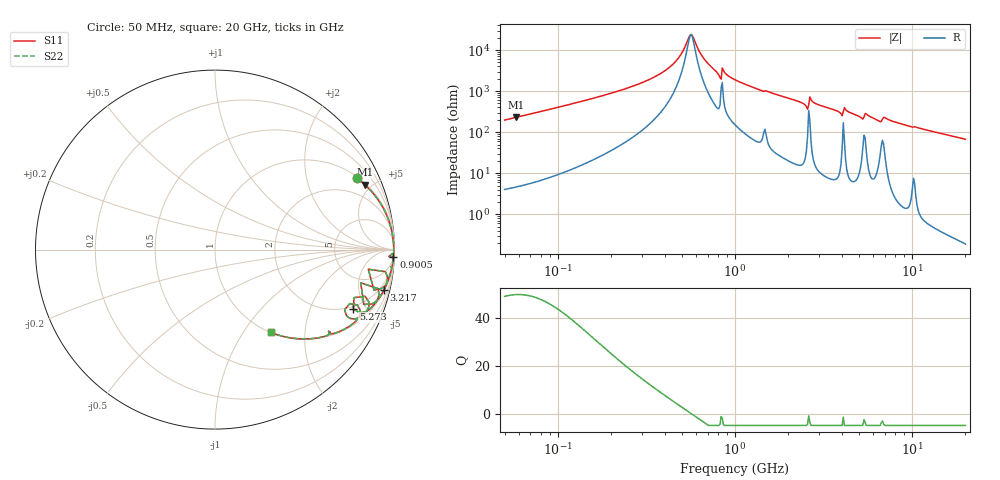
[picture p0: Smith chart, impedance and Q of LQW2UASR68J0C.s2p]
!Murata Part Number: LQW2UASR68J0C
!These Parameters are Measured in Series Mode Connection
!  o--[Z]--o
!Port1  Port2
!  o-------o
!Freq. Start=50[MHz] Stop=20[GHz], 401[Steps]
# Hz S RI R 50
!Freq.(Hz) S11(Real) S11(Imag) S21(Real) S21(Imag) S12(Real) S12(Imag) S22(Real) S22(Imag)
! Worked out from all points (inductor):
!   401 points, 50 MHz to 20 GHz, reference 50 ohm
!   read as one part in series: L = 621 nH near 51.52 MHz
!   highest Q = 49.8 at 58.08 MHz (marker M1), where L = 628 nH
!   self-resonance near 557.6 MHz
!   S11 on the Smith chart (normalised r, x): 50 MHz: 1.08, +3.94; 900.5 MHz: 7, -49; 3.217 GHz: 1.17, -8.26; 5.273 GHz: 1.84, -4.09; 20 GHz: 1.00, -1.34
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5e7  0.7903 0.397  0.2097 -0.397  0.2097 -0.397  0.7903 0.397
5.807932e7  0.8353 0.361  0.1647 -0.361  0.1647 -0.361  0.8353 0.361
1.364002e8  0.9652 0.1699  0.0348 -0.1699  0.0348 -0.1699  0.9652 0.1699
2.520729e8  0.9892 0.0803  0.0108 -0.0803  0.0108 -0.0803  0.9892 0.0803
3.721004e8  0.9943 0.0387  0.00569 -0.0387  0.00569 -0.0387  0.9943 0.0387
4.658406e8  0.9955 0.0175  0.00446 -0.0175  0.00446 -0.0175  0.9955 0.0175
5.659842e8  0.9959 -0.000196  0.00414 0.000196  0.00414 0.000196  0.9959 -0.000196
6.574395e8  0.9956 -0.014  0.00435 0.014  0.00435 0.014  0.9956 -0.014
8.108264e8  0.9924 -0.0394  0.00762 0.0394  0.00762 0.0394  0.9924 -0.0394
8.738837e8  0.9936 -0.0344  0.00636 0.0344  0.00636 0.0344  0.9936 -0.0344
9.00459e8  0.9939 -0.0395  0.00607 0.0395  0.00607 0.0395  0.9939 -0.0395
1e9  0.9931 -0.0521  0.00693 0.0521  0.00693 0.0521  0.9931 -0.0521
2.493527e9  0.9451 -0.2038  0.0549 0.2038  0.0549 0.2038  0.9451 -0.2038
2.728004e9  0.961 -0.1682  0.039 0.1682  0.039 0.1682  0.961 -0.1682
3.216634e9  0.9405 -0.2266  0.0595 0.2266  0.0595 0.2266  0.9405 -0.2266
3.908127e9  0.8922 -0.2928  0.1078 0.2928  0.1078 0.2928  0.8922 -0.2928
4.212059e9  0.9135 -0.2526  0.0865 0.2526  0.0865 0.2526  0.9135 -0.2526
5.273168e9  0.7706 -0.3301  0.2294 0.3301  0.2294 0.3301  0.7706 -0.3301
5.683258e9  0.8518 -0.3318  0.1482 0.3318  0.1482 0.3318  0.8518 -0.3318
7.442007e9  0.7894 -0.3932  0.2106 0.3932  0.2106 0.3932  0.7894 -0.3932
1.201863e10  0.5625 -0.4933  0.4375 0.4933  0.4375 0.4933  0.5625 -0.4933
2e10  0.3117 -0.4618  0.6883 0.4618  0.6883 0.4618  0.3117 -0.4618
